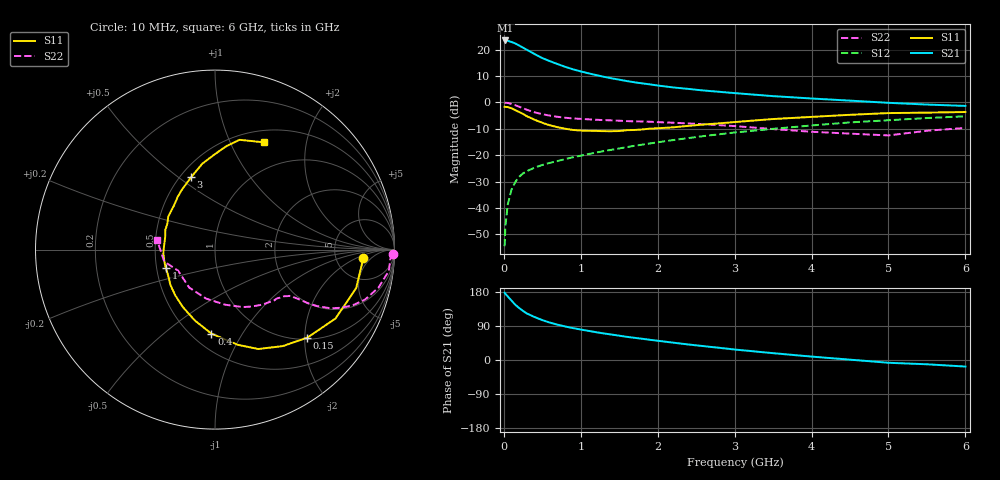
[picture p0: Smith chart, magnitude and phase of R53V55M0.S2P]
! SIEMENS Small Signal Semiconductors
! BFR183
! Si NPN RF Bipolar Junction Transistor in SOT23
! VCE = 3.5 V  IC = 5 mA
! Common Emitter S-Parameters:  May  1996
# GHz  S  MA  R  50
!  f  S11  S21  S12  S22
! GHz  MAG  ANG  MAG  ANG  MAG  ANG  MAG  ANG
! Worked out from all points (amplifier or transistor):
!   36 points, 10 MHz to 6 GHz, reference 50 ohm
!   highest |S21| = 23.4 dB at 20 MHz (marker M1)
!   |S21| within 3 dB of that: start of sweep to 265.9 MHz
!   unconditionally stable (mu >= 1): 1.048 GHz to 2.644 GHz
!   at 250 MHz: K = 0.41, MSG = 23.8 dB, |S12| = -26.9 dB
!   at 1.4 GHz: K = 1.06, MAG = 12.0 dB, |S12| = -18.0 dB
!   at 6 GHz: K = 0.88, MSG = 2.0 dB, |S12| = -5.3 dB
!   lowest NFmin = 1.15 dB at 450 MHz
!   S11 on the Smith chart (normalised r, x): 10 MHz: 10, -3; 150 MHz: 1.04, -2.06; 400 MHz: 0.62, -0.74; 1 GHz: 0.56, -0.12; 3 GHz: 0.57, +0.56; 6 GHz: 0.64, +1.35
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0.01  0.827 -3.2  14.67 177.7  0.0019 92.8  0.9902 -1.3
0.02  0.8217 -6.1  14.84 174.9  0.0045 87.5  0.9789 -2.8
0.05  0.8151 -15.3  14.63 167.9  0.0115 81.7  0.9757 -7.0
0.1  0.7735 -29.8  13.88 156.7  0.0224 75.2  0.9351 -13.1
0.15  0.7103 -43.7  13.02 145.5  0.0314 68.9  0.8811 -18.4
0.2  0.6571 -54.9  11.88 137.1  0.0392 65.0  0.8266 -22.1
0.25  0.6039 -66.5  10.81 129.3  0.0453 60.9  0.7728 -24.8
0.3  0.5456 -76.5  9.875 122.7  0.0501 59.1  0.7232 -26.9
0.4  0.4687 -92.4  8.202 113.4  0.0581 56.5  0.6481 -29.0
0.5  0.4107 -105.9  6.888 105.2  0.0653 55.1  0.5969 -30.0
0.6  0.3676 -118.9  6.007 98.6  0.0717 55.7  0.5603 -30.4
0.7  0.3382 -130.7  5.293 93.1  0.0778 55.9  0.5326 -30.8
0.8  0.3169 -141.8  4.694 88.3  0.0845 56.2  0.5115 -31.2
1  0.2927 -159.6  3.849 80.3  0.098 57.5  0.4868 -32.0
1.1  0.2899 -167.3  3.546 76.9  0.105 57.9  0.4777 -32.9
1.6  0.2977 158.5  2.529 61.1  0.1425 58.9  0.442 -37.8
2.2  0.3368 132.4  1.918 45.8  0.1933 57.1  0.412 -46.8
3  0.424 108.4  1.497 27.7  0.269 51.0  0.3557 -64.2
3.5  0.4839 98.4  1.312 18.0  0.3158 45.6  0.3123 -79.5
4.5  0.5815 83.5  1.078 0.9  0.4178 33.8  0.256 -124.1
5.5  0.6395 70.9  0.909 -11.3  0.5049 21.3  0.2903 -166.7
6  0.6568 65.4  0.857 -17.3  0.5452 13.1  0.3283 170.3
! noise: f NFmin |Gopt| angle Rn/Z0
0.45  1.15  0.25  40  0.26
0.9  1.2  0.25  93  0.22
1.8  1.95  0.32  170  0.13
